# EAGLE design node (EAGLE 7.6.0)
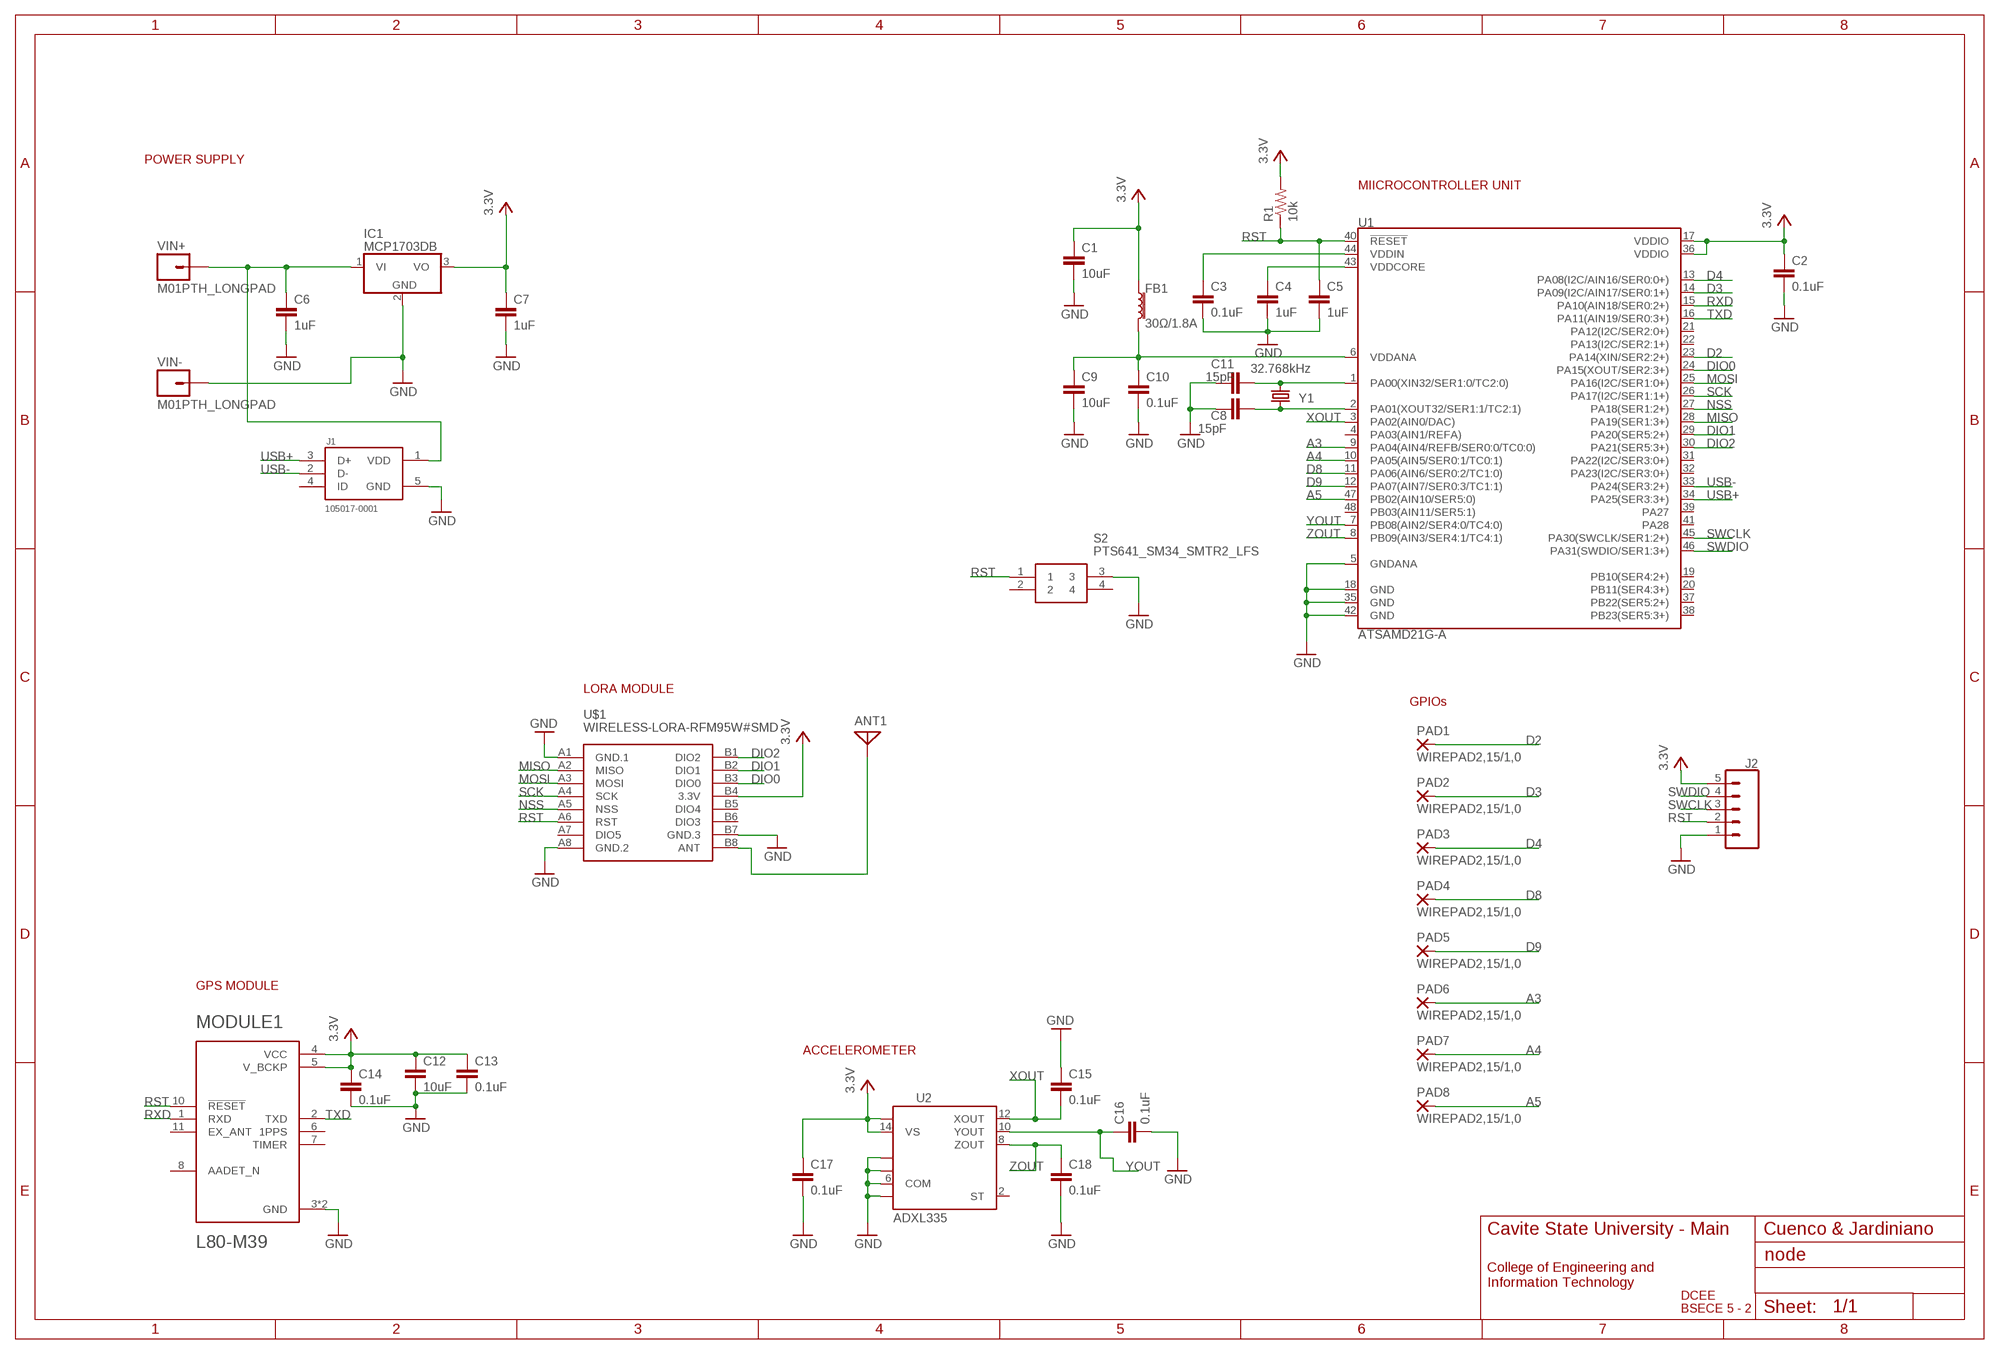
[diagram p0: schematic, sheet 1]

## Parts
ANT1  ANTENNA  [PAD-01]
C1  10uF  10UF-1206-6.3V-20%  [1206]
C2  0.1uF  10UF-1206-6.3V-20%  [1206]
C3  0.1uF  10UF-1206-6.3V-20%  [1206]
C4  1uF  10UF-1206-6.3V-20%  [1206]
C5  1uF  10UF-1206-6.3V-20%  [1206]
C6  1uF  10UF-1206-6.3V-20%  [1206]
C7  1uF  10UF-1206-6.3V-20%  [1206]
C8  15pF  10UF-1206-6.3V-20%  [1206]
C9  10uF  10UF-1206-6.3V-20%  [1206]
C10  0.1uF  10UF-1206-6.3V-20%  [1206]
C11  15pF  10UF-1206-6.3V-20%  [1206]
C12  10uF  10UF-1206-6.3V-20%  [1206]
C13  0.1uF  10UF-1206-6.3V-20%  [1206]
C14  0.1uF  10UF-1206-6.3V-20%  [1206]
C15  0.1uF  10UF-1206-6.3V-20%  [1206]
C16  0.1uF  10UF-1206-6.3V-20%  [1206]
C17  0.1uF  10UF-1206-6.3V-20%  [1206]
C18  0.1uF  10UF-1206-6.3V-20%  [1206]
FB1  30Ω/1.8A  FERRITE_BEAD-0603  [0603]
IC1  MCP1703DB  [SOT223]
J1  105017-0001  [MOLEX_105017-0001]
J2  CONN_05  [1X05]
MODULE1  L80-M39  [QUECTEL_L80-M39]
PAD1  WIREPAD2,15/1,0  [2,15/1,0]
PAD2  WIREPAD2,15/1,0  [2,15/1,0]
PAD3  WIREPAD2,15/1,0  [2,15/1,0]
PAD4  WIREPAD2,15/1,0  [2,15/1,0]
PAD5  WIREPAD2,15/1,0  [2,15/1,0]
PAD6  WIREPAD2,15/1,0  [2,15/1,0]
PAD7  WIREPAD2,15/1,0  [2,15/1,0]
PAD8  WIREPAD2,15/1,0  [2,15/1,0]
R1  10k  RESISTOR1206  [1206]
S2  PTS641_SM34_SMTR2_LFS  [PTS641_SM34]
U1  ATSAMD21G-A  [TQFP-48]
U2  ADXL335  [LFCSP-16]
U$1  WIRELESS-LORA-RFM95W#SMD  [WIRELESS-LORA-RFM95W#SMD]
VIN+  M01PTH_LONGPAD  [1X01_LONGPAD]
VIN-  M01PTH_LONGPAD  [1X01_LONGPAD]
Y1  32.768kHz  CRYSTAL-32.768KHZSMD-3.2X1.5  [CRYSTAL-SMD-3.2X1.5MM]

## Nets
A3: PAD6.1(P) U1.9(PA04(AIN4/REFB/SER0:0/TC0:0))
A4: PAD7.1(P) U1.10(PA05(AIN5/SER0:1/TC0:1))
A5: PAD8.1(P) U1.47(PB02(AIN10/SER5:0))
D2: PAD1.1(P) U1.23(PA14(XIN/SER2:2+))
D3: PAD2.1(P) U1.14(PA09(I2C/AIN17/SER0:1+))
D4: PAD3.1(P) U1.13(PA08(I2C/AIN16/SER0:0+))
D8: PAD4.1(P) U1.11(PA06(AIN6/SER0:2/TC1:0))
D9: PAD5.1(P) U1.12(PA07(AIN7/SER0:3/TC1:1))
DIO0: U1.24(PA15(XOUT/SER2:3+)) U$1.B3(DIO0)
DIO1: U1.29(PA20(SER5:2+)) U$1.B2(DIO1)
DIO2: U1.30(PA21(SER5:3+)) U$1.B1(DIO2)
FB1: C9.1 C10.1 FB1.2 U1.6(VDDANA)
GND: C1.2 C2.2 C3.2 C4.2 C5.2 C6.2 C7.2 C8.2 C9.2 C10.2 C11.1 C12.2 C13.2 C14.2 C15.1 C16.2 C17.2 C18.2 IC1.2(GND) J1.5(GND) J2.1 MODULE1.3(GND) MODULE1.12(GND) S2.3 U1.5(GNDANA) U1.18(GND) U1.35(GND) U1.42(GND) U2.3(COM) U2.5(COM) U2.6(COM) U2.7(COM) U$1.A1(GND.1) U$1.A8(GND.2) U$1.B7(GND.3) VIN-.1
MISO: U1.28(PA19(SER1:3+)) U$1.A2(MISO)
MOSI: U1.25(PA16(I2C/SER1:0+)) U$1.A3(MOSI)
N$1: C8.1 U1.1(PA00(XIN32/SER1:0/TC2:0)) Y1.P$2
N$2: C11.2 U1.2(PA01(XOUT32/SER1:1/TC2:1)) Y1.P$1
N$3: C4.1 U1.43(VDDCORE)
N$4: ANT1.1 U$1.B8(ANT)
N$5: C6.1 IC1.1(VI) J1.1(VDD) VIN+.1
N$6: C3.1 U1.44(VDDIN)
NSS: U1.27(PA18(SER1:2+)) U$1.A5(NSS)
RST: C5.1 J2.2 MODULE1.10(!RESET) R1.1 S2.1 U1.40(!RESET!) U$1.A6(RST)
RXD: MODULE1.1(RXD) U1.15(PA10(AIN18/SER0:2+))
SCK: U1.26(PA17(I2C/SER1:1+)) U$1.A4(SCK)
SWCLK: J2.3 U1.45(PA30(SWCLK/SER1:2+))
SWDIO: J2.4 U1.46(PA31(SWDIO/SER1:3+))
TXD: MODULE1.2(TXD) U1.16(PA11(AIN19/SER0:3+))
USB+: J1.3(D+) U1.34(PA25(SER3:3+))
USB-: J1.2(D-) U1.33(PA24(SER3:2+))
VCC: C1.1 C2.1 C7.1 C12.1 C13.1 C14.1 C17.1 FB1.1 IC1.3(VO) J2.5 MODULE1.4(VCC) MODULE1.5(V_BCKP) R1.2 U1.17(VDDIO) U1.36(VDDIO) U2.14(VS) U2.15(VS) U$1.B4(3.3V) ; supply symbol labelled 3.3V
XOUT: C15.2 U1.3(PA02(AIN0/DAC)) U2.12(XOUT)
YOUT: C16.1 U1.7(PB08(AIN2/SER4:0/TC4:0)) U2.10(YOUT)
ZOUT: C18.1 U1.8(PB09(AIN3/SER4:1/TC4:1)) U2.8(ZOUT)
Unconnected: J1.4(ID) MODULE1.6(1PPS) MODULE1.7(TIMER) MODULE1.8(AADET_N) MODULE1.11(EX_ANT) S2.2 S2.4 U1.4(PA03(AIN1/REFA)) U1.19(PB10(SER4:2+)) U1.20(PB11(SER4:3+)) U1.21(PA12(I2C/SER2:0+)) U1.22(PA13(I2C/SER2:1+)) U1.31(PA22(I2C/SER3:0+)) U1.32(PA23(I2C/SER3:0+)) U1.37(PB22(SER5:2+)) U1.38(PB23(SER5:3+)) U1.39(PA27) U1.41(PA28) U1.48(PB03(AIN11/SER5:1)) U2.2(ST) U$1.A7(DIO5) U$1.B5(DIO4) U$1.B6(DIO3)

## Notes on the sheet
- POWER SUPPLY
- MIICROCONTROLLER UNIT
- LORA MODULE
- GPIOs
- GPS MODULE
- ACCELEROMETER
- Cavite State University - Main | Cuenco & Jardiniano
- College of Engineering and
  Information Technology
- DCEE
- BSECE 5 - 2

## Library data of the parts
ANT1 = discrete:ANTENNA: Antenna
C1 C9 C12 = SparkFun-Capacitors:10UF: 10.0µF ceramic capacitors; PROD_ID: CAP-10057
C2-C8 C10 C11 C13-C18 = SparkFun-Capacitors:10UF: 10.0µF ceramic capacitors; PROD_ID: CAP-10057; VALUE: 10uF
FB1 = SparkFun-Coils:FERRITE_BEAD: Ferrite Bead (blocks, cores, rings, chokes, etc.); PROD_ID: NDUC-13805
IC1 = linear (1):MCP1703: 250 mA, 16V, Low Quiescent Current LDO Regulator Source: http://ww1.microchip.com/downloads/en/DeviceDoc/22049b.pdf
J1 = 105017-0001:105017-0001; AVAILABILITY: Unavailable; DESCRIPTION: Conn USB Type B M 5 POS 0.65mm Solder RA Thru-Hole 5 Terminal 1 Port Embossed T/R; MF: Molex, LLC; MP: 105017-0001; PACKAGE: None; PRICE: None
J2 = SparkFun-Connectors:CONN_05: Multi connection point. Often used as Generic Header-pin footprint for 0.1 inch spaced/style header connections On any of the 0.1 inch spaced packages, you can populate with these: Break Away Headers - Straight (PRT-00116) Break Away Male Headers - Right Angle (PRT-00553) Female Headers (PRT-00115)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
MODULE1 = L80-M39:L80-M39: GPS Receiver 1575.42MHz 3.3V 12-Pin; AVAILABILITY: Unavailable; DESCRIPTION: GPS Receiver 1575.42MHz 3.3V 12-Pin; MF: Quectel; MP: L80-M39; PACKAGE: None; PRICE: None
PAD1-PAD8 = wirepad:WIREPAD: Wire PAD connect wire on PCB
R1 = SparkFun:RESISTOR: Resistor
S2 = PTS641_SM34_SMTR2_LFS:PTS641_SM34_SMTR2_LFS: PTS641 Series SMT Top Actuated Switches Source: Datasheet; DESCRIPTION: PTS641 Series SMT Top Actuated Switches; HEIGHT: mm; MANUFACTURER_NAME: C & K COMPONENTS; MANUFACTURER_PART_NUMBER: PTS641 SM34 SMTR2 LFS; MOUSER_PART_NUMBER: 1359404P; MOUSER_PRICE-STOCK: http://uk.rs-online.com/web/p/products/1359404P; RS_PART_NUMBER: 1359404P; RS_PRICE-STOCK: http://uk.rs-online.com/web/p/products/1359404P
U1 = SparkFun-IC-Microcontroller:ATSAMD21G: Atmel SAMD21G SMART ARM-Based Microcontroller The Atmel ® | SMART ™ SAM D21 is a series of low-power microcontrollers using the 32-bit ARM ® Cortex ® -M0+ processor, and ranging from 32- to 64-pins with up to 256KB Flash and 32KB of SRAM. The SAM D21 devices operate at a maximum frequency of 48MHz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; PROD_ID: IC-13064
U2 = SparkFun:ADXL335
U$1 = diy-modules:WIRELESS-LORA-RFM95W: 868/915 MHz LoRa Radio Transceiver Module based on SX1276 chip Click here to find device on ebay.com
VIN+ VIN- = SparkFun:M01: Header 1
Y1 = SparkFun-Clocks:CRYSTAL-32.768KHZ: 32.768kHz Crystal; PROD_ID: XTAL-13062

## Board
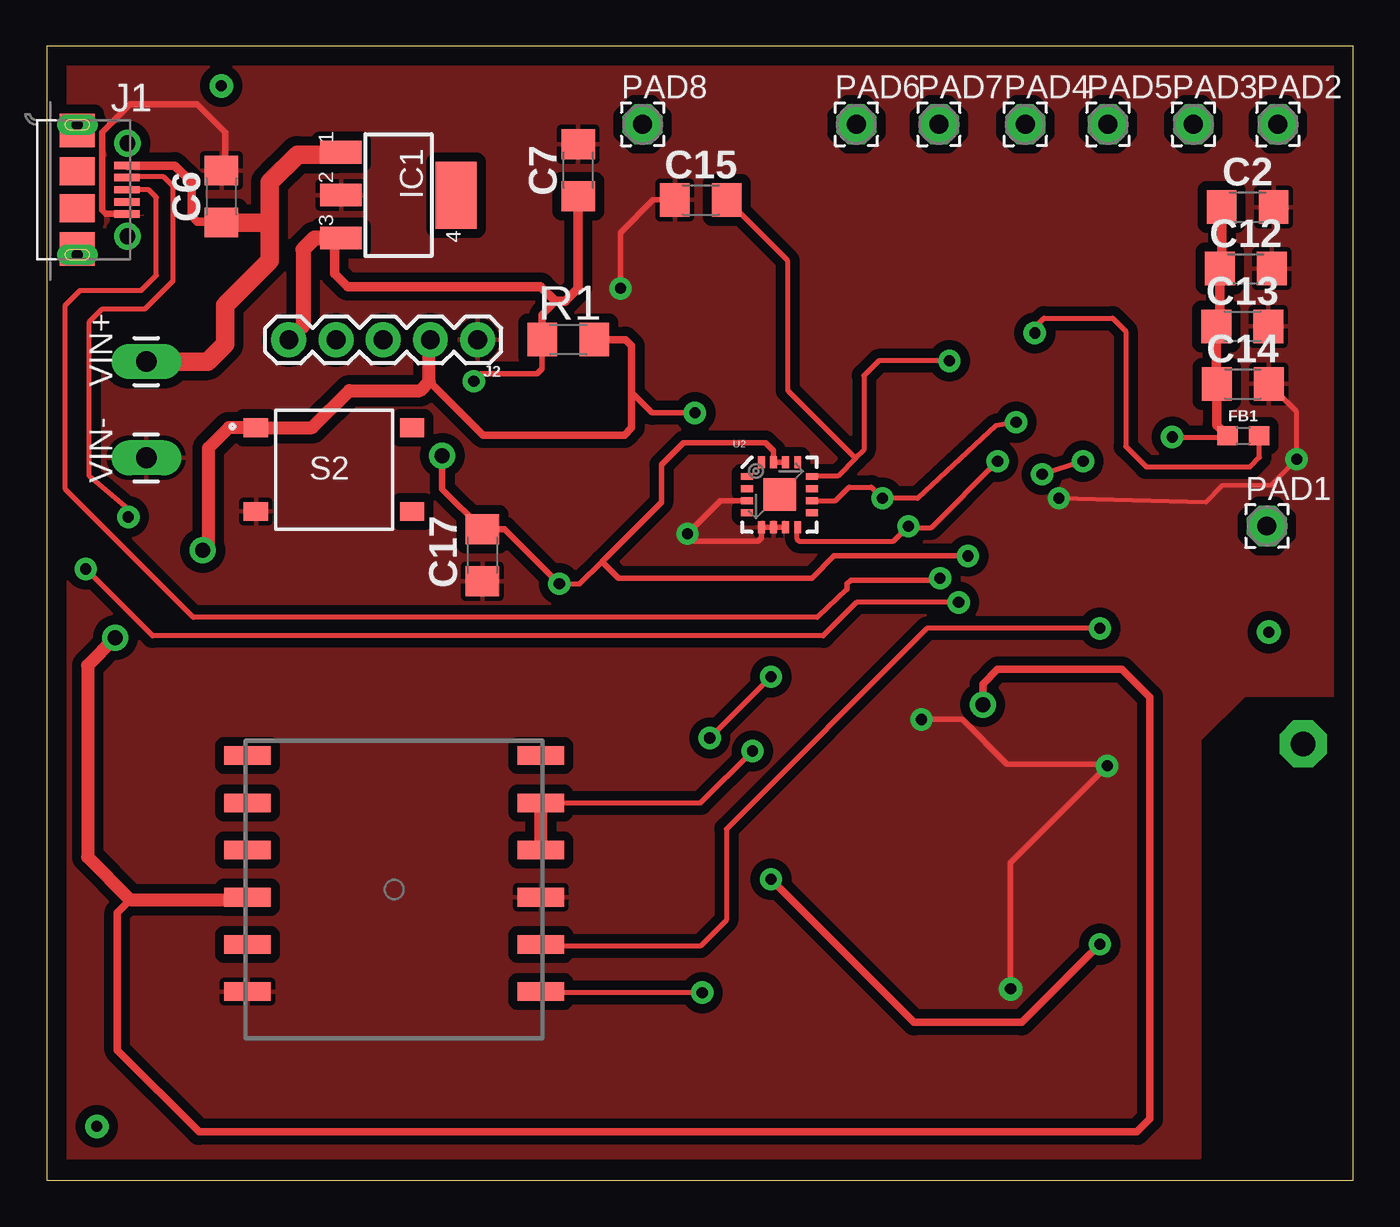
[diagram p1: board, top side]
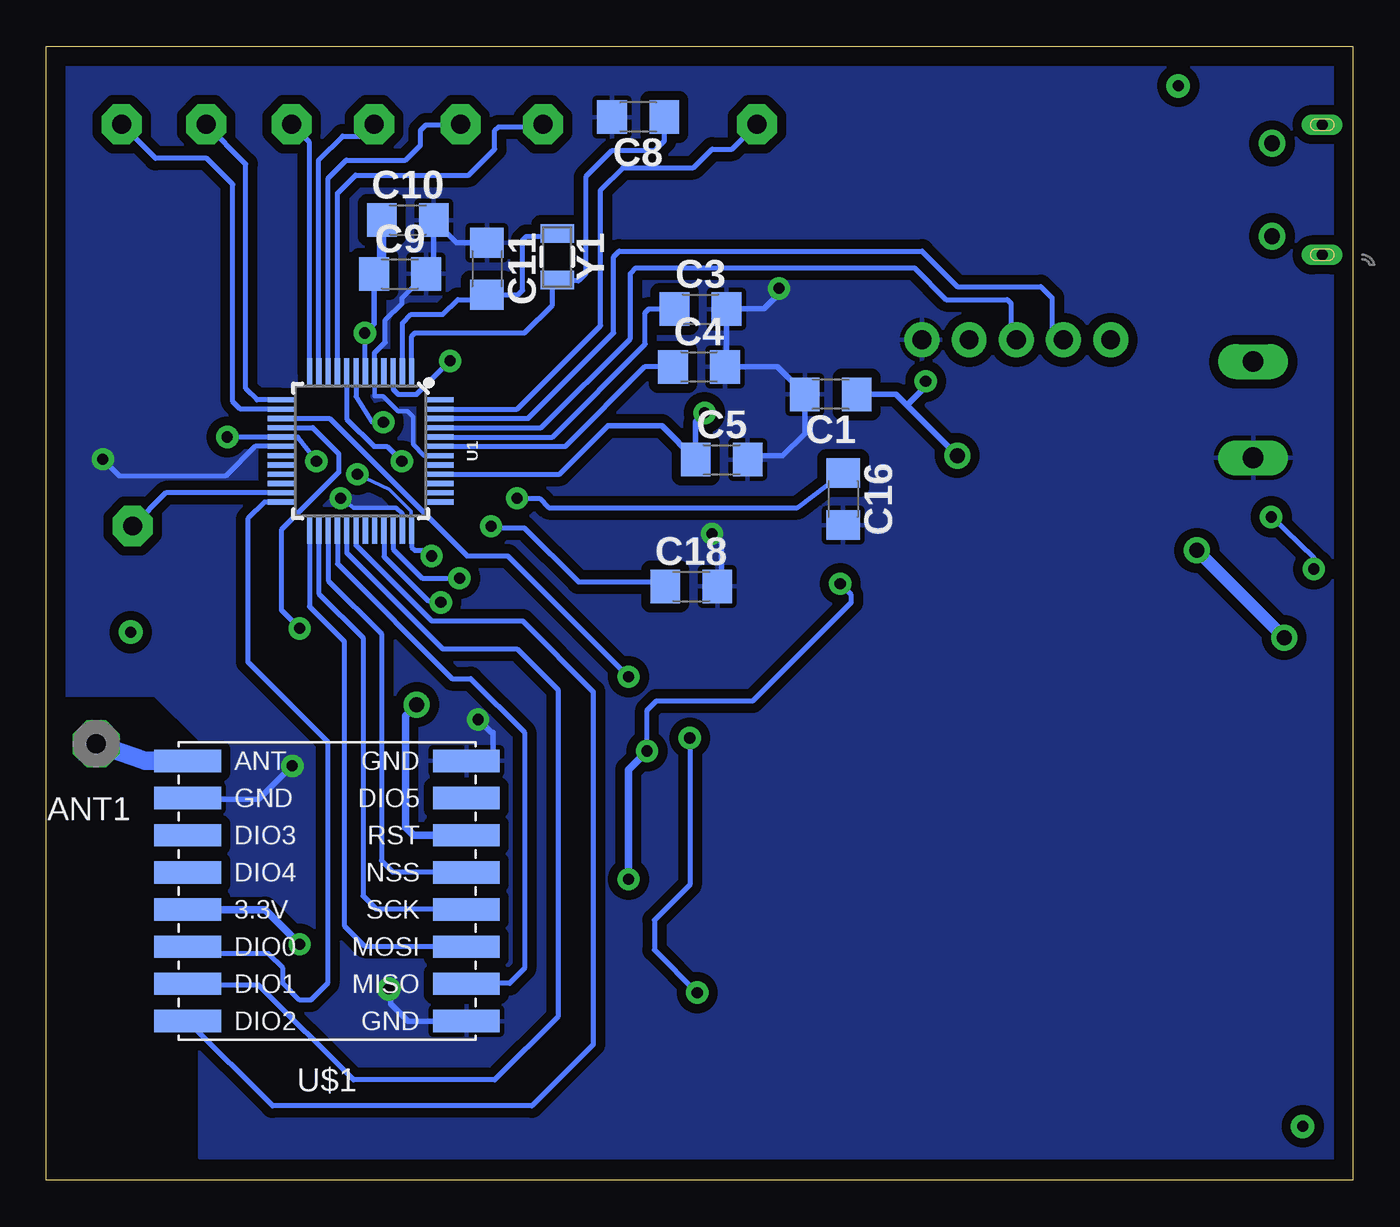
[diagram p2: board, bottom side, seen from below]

Size 70.34 x 61.02 mm. Coordinates in mm from the lower left corner, seen from the top.
Outline: 0,0 70.34,0 70.34,61.02 0,61.02 0,0
Copper layers (1*16): Top 0.035mm / dielectric 1.5mm / Bottom 0.035mm
Design rules "default *": minimum track width 4mil, minimum drill 16mil, track to track 8mil, track to pad 8mil, pad to pad 8mil, via to via 8mil, smd to smd 8mil, copper to edge 40mil, drill to drill 8mil, minimum pad ring 10mil, minimum via ring 8mil, stop-mask expansion 4mil, vias tented up to drill 0mil, thermal gap 10mil

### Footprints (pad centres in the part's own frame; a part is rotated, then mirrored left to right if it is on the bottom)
PAD-01 = drill 1.321 pad 2.54 octagon: 1 0,0
1206 = smd 1.6 x 1.8: 1 -1.4,0; 2 1.4,0
0603 = smd 1.1 x 1: 1 -0.85,0; 2 0.85,0
SOT223 = smd 1.219 x 2.235: 1 -2.311,-3.099; 2 0,-3.099; 3 2.311,-3.099 | smd 3.6 x 2.2: 4 0,3.099
MOLEX_105017-0001 = smd 0.4 x 1.35: 1 -1.3,2.675; 2 -0.65,2.675; 3 0,2.675; 4 0.65,2.675; 5 1.3,2.675 | drill 0.85 pad 1.45: P$1 -2.5,2.7; P$2 2.5,2.7 | smd 1.5 x 1.9: P$8 -1,0; P$9 1,0 | smd 1.8 x 1.9: P$10 -3.2,0; P$11 3.2,0 | drill 0.6 pad 0.8 long: P$12 -3.5,0; P$13 3.5,0
1X05 = drill 1.016 pad 1.88: 1 0,0; 2 2.54,0; 3 5.08,0; 4 7.62,0; 5 10.16,0
QUECTEL_L80-M39 = smd 2.5 x 1: 1 7.9,-5.5; 2 7.9,-2.96; 3 7.9,-0.42; 4 7.9,2.12; 5 7.9,4.66; 6 7.9,7.2; 7 -7.9,7.2; 8 -7.9,4.66; 9 -7.9,2.12; 10 -7.9,-0.42; 11 -7.9,-2.96; 12 -7.9,-5.5
2,15/1,0 = drill 1.016 pad 2.159 octagon: 1 0,0
PTS641_SM34 = smd 1.3 x 1: 1 -4.2,2.25; 2 4.2,2.25; 3 -4.2,-2.25; 4 4.2,-2.25
TQFP-48 = smd 1.5 x 0.28: 1 -4.25,2.75; 2 -4.25,2.25; 3 -4.25,1.75; 4 -4.25,1.25; 5 -4.25,0.75; 6 -4.25,0.25; 7 -4.25,-0.25; 8 -4.25,-0.75; 9 -4.25,-1.25; 10 -4.25,-1.75; 11 -4.25,-2.25; 12 -4.25,-2.75; 25 4.25,-2.75; 26 4.25,-2.25; 27 4.25,-1.75; 28 4.25,-1.25; 29 4.25,-0.75; 30 4.25,-0.25; 31 4.25,0.25; 32 4.25,0.75; 33 4.25,1.25; 34 4.25,1.75; 35 4.25,2.25; 36 4.25,2.75 | smd 0.28 x 1.5: 13 -2.75,-4.25; 14 -2.25,-4.25; 15 -1.75,-4.25; 16 -1.25,-4.25; 17 -0.75,-4.25; 18 -0.25,-4.25; 19 0.25,-4.25; 20 0.75,-4.25; 21 1.25,-4.25; 22 1.75,-4.25; 23 2.25,-4.25; 24 2.75,-4.25; 37 2.75,4.25; 38 2.25,4.25; 39 1.75,4.25; 40 1.25,4.25; 41 0.75,4.25; 42 0.25,4.25; 43 -0.25,4.25; 44 -0.75,4.25; 45 -1.25,4.25; 46 -1.75,4.25; 47 -2.25,4.25; 48 -2.75,4.25
LFCSP-16 = smd 1.75 x 1.75: 0 0,0 | smd 0.65 x 0.37: 1 -1.75,0.975; 2 -1.75,0.325; 3 -1.75,-0.325; 4 -1.75,-0.975; 9 1.75,-0.975; 10 1.75,-0.325; 11 1.75,0.325; 12 1.75,0.975 | smd 0.37 x 0.65: 5 -0.975,-1.75; 6 -0.325,-1.75; 7 0.325,-1.75; 8 0.975,-1.75; 13 0.975,1.75; 14 0.325,1.75; 15 -0.325,1.75; 16 -0.975,1.75
WIRELESS-LORA-RFM95W#SMD = smd 3.6 x 1.2: A1 -7.5,7; A2 -7.5,5; A3 -7.5,3; A4 -7.5,1; A5 -7.5,-1; A6 -7.5,-3; A7 -7.5,-5; A8 -7.5,-7; B1 7.5,7; B2 7.5,5; B3 7.5,3; B4 7.5,1; B5 7.5,-1; B6 7.5,-3; B7 7.5,-5; B8 7.5,-7
1X01_LONGPAD = drill 1.118 pad 1.88 long: 1 0,0
CRYSTAL-SMD-3.2X1.5MM = smd 1 x 1.8: P$1 -1.25,0; P$2 1.25,0

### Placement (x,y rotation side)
ANT1  67.65,23.49 180 bottom
C1  28.11,42.3 180 bottom
C2  64.66,52.38 0 top
C3  35.12,46.88 0 bottom
C4  35.2,43.78 0 bottom
C5  33.98,38.78 0 bottom
C6  9.42,52.94 90 top
C7  28.62,54.36 90 top
C8  38.48,57.22 180 bottom
C9  51.3,48.78 0 bottom
C10  50.88,51.68 0 bottom
C11  46.62,49.06 270 bottom
C12  64.56,49.06 0 top
C13  64.38,45.96 0 top
C14  64.4,42.86 0 top
C15  35.22,52.76 0 top
C16  27.44,36.66 270 bottom
C17  23.46,33.64 270 top
C18  35.62,31.96 0 bottom
FB1  64.42,40.07 0 top
IC1  18.94,53.02 270 top
J1  1.65,53.31 270 top
J2  23.2,45.23 180 top
MODULE1  18.71,15.65 0 top
PAD1  65.7,35.21 0 top
PAD2  66.29,56.83 0 top
PAD3  61.74,56.83 0 top
PAD4  52.69,56.83 0 top
PAD5  57.14,56.83 0 top
PAD6  43.59,56.83 0 top
PAD7  48.04,56.83 0 top
PAD8  32.09,56.83 0 top
R1  28.08,45.24 180 top
S2  15.47,38.25 0 top
U1  53.42,39.25 270 bottom
U2  39.46,36.9 0 top
U$1  55.23,15.57 180 bottom
VIN+  5.37,44.06 90 top
VIN-  5.37,38.88 90 top
Y1  42.84,49.7 270 bottom

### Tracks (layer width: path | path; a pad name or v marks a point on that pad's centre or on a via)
A3
  Bottom 0.279: U1.9 54.67,53.13 53.7,54.1 47.6,54.1 46.2,55.5 46.2,56.5 46,56.7 43.72,56.7 PAD6.1
A4
  Bottom 0.279: U1.10 55.17,53.93 54.2,54.9 51,54.9 50.2,55.7 50.2,56.5 49.9,56.8 48.07,56.8 PAD7.1
A5
  Bottom 0.279: U1.47 45,41.5 40.5,46 40.5,53.3 39.3,54.5 35.5,54.5 34.5,55.5 33.42,55.5 PAD8.1
D2
  Bottom 0.279: U1.23 63.91,37 PAD1.1
D3
  Bottom 0.279: U1.14 59.9,41.5 60.3,41.9 60.3,53.6 61.7,55 64.46,55 PAD2.1
D4
  Bottom 0.279: U1.13 59,42 59.6,42.6 59.6,54.69 PAD3.1
D8
  Bottom 0.279: U1.11 55.67,54.93 54.4,56.2 53.32,56.2 PAD4.1
D9
  Bottom 0.279: U1.12 56.17,55.86 PAD5.1
DIO0
  Bottom 0.279: U1.24 58.6,36.5 59.5,35.6 59.5,27.9 55.2,23.6 55.2,10.6 56.1,9.7 56.7,9.7 57.6,10.6 57.6,11.4 58.4,12.2 62.36,12.2 U$1.B3
DIO1
  Bottom 0.279: U1.29 54.17,33.77 49,28.6 45,28.6 42.8,26.4 42.8,8.8 46.2,5.4 53.8,5.4 58.9,10.5 62.66,10.5 U$1.B2
DIO2
  Bottom 0.279: U1.30 53.67,34.17 49.6,30.1 44.7,30.1 40.9,26.3 40.9,7.3 44.2,4 58.16,4 U$1.B1
FB1  (via drill 0.6 pad 1.2)
  Top 0.279: v53.2,45.6 53.2,45.9 53.7,46.4 57.4,46.4 58.1,45.7 58.1,39.5 59.2,38.4 64.8,38.4 65.3,38.9 65.3,40.04 FB1.2
  Bottom 0.279: U1.6 53.17,45.57 v53.2,45.6
  Bottom 0.3: C9.1 52.7,46.1 v53.2,45.6
  Bottom 0.5: C10.1 52.28,49.2 C9.1
GND  (via drill 0.6 pad 1.2, 0.6 pad 1.27)
  Top 0.25: v54.5,36.7 62.4,36.5 63.3,37.4 65.9,37.4 v67.3,38.8
  Top 0.279: v67.3,38.8 67.3,41.36 C14.2
  Top 0.3: U2.7 U2.6 U2.5 38.48,34.59 38.3,34.4 34.9,34.4 v34.5,34.8 36.27,36.58 U2.3 | C15.1 32.66,52.76 30.9,51 v30.9,48 | v47.1,24.8 49.3,24.8 51.7,22.4 57,22.4 v57.1,22.3 51.9,17.1 v51.9,10.3
  Top 0.35: J1.5 3.19,52.01 3,52.2 3,56.4 4.5,57.9 8.1,57.9 9.6,56.4 9.6,54.52 C6.2
  Bottom 0.25: U1.42 50,39 50.6,39.6 50.6,41.1 50.9,41.4 51.4,41.4 52.2,42.2 52.67,42.2 U1.5 | U1.35 51.17,35.87 51.5,36.2 53.8,36.2 v54.5,36.7
  Bottom 0.279: U1.5 52.67,44.53 52.1,45.1 52.1,46.3 51.2,47.2 51.2,47.48 C9.2 | U1.18 59.1,39.5 60.7,37.9 66.4,37.9 v67.3,38.8
  Bottom 0.3: C9.2 49.48,49.2 C10.2 48.26,50.46 C11.1 | v34.5,34.8 34,34.3 34,32.18 C18.2 | C5.2 32.36,39 30.7,39 29.51,40.19 C1.2 30.99,43.78 C4.2 33.72,43.86 C3.2 33.7,46.9 31.7,46.9 30.9,47.7 v30.9,48 | U$1.A8 46.3,22.57 46.3,24.1 46.4,24.1 v47.1,24.8 | v57.1,22.3 58.9,20.5 62.66,20.5 U$1.B7 | U$1.A1 50.87,8.57 51.8,9.5 51.8,10.2 v51.9,10.3
  pour Top (isolate 0.5): 0.9,60.3 69.6,60.3 69.6,26.1 64.5,26.1 62.1,23.7 62.1,1.2 0.9,1.2
  pour Bottom (isolate 0.5): 0.9,60.3 69.6,60.3 69.6,26.1 64.5,26.1 62.1,23.7 62.1,1.2 0.9,1.2
MISO
  Bottom 0.279: U1.28 54.67,33.17 48.5,27 47.5,27 44.6,24.1 44.6,11.4 45.4,10.6 47.7,10.6 U$1.A2
MOSI
  Bottom 0.279: U1.25 56.17,30.87 54.3,29 54.3,13.7 53.2,12.6 47.76,12.6 U$1.A3
N$1
  Bottom 0.279: U1.1 50.67,45.43 50.5,45.6 44.6,45.6 43.1,47.1 43.1,48.19 Y1.P$2 42.79,48.4 41.7,48.4 41.3,48.8 41.3,54 39.9,55.4 37.6,55.4 37.08,55.92 C8.1
N$2
  Bottom 0.279: U1.2 51.17,46.13 50.7,46.6 49,46.6 48.2,47.4 46.98,47.4 C11.2 44.94,47.66 44.7,47.9 44.7,50.6 44.5,50.8 42.99,50.8 Y1.P$1
N$3
  Bottom 0.279: U1.43 42.4,39.5 38.1,43.8 36.62,43.8 C4.1
N$4
  Bottom 1: U$1.B8 65.03,22.57 ANT1.1
N$5
  Top 0.45: J1.1 6.89,54.61 7.8,53.7 7.8,51.9 8.1,51.6 9.36,51.6 C6.1
  Top 1: VIN+.1 8.66,44.06 9.6,45 9.6,47.1 12,49.5 12,51.6 | 12,51.6 12,53.7 13.5,55.2 15.71,55.2 IC1.1 | C6.1 11.94,51.54 12,51.6
N$6
  Bottom 0.279: U1.44 43.1,40 38.1,45 38.1,46.7 37.9,46.9 36.54,46.9 C3.1
N$7  (via drill 0.6 pad 1.27)
  other vias: 2.7,2.9
N$8  (via drill 0.6 pad 1.27)
  other vias: 9.4,58.9
N$14  (via drill 0.6 pad 1.27)
  other vias: 65.8,29.5
NSS
  Bottom 0.279: U1.27 55.17,32.27 52.3,29.4 52.3,17.2 51.7,16.6 47.76,16.6 U$1.A5
RST  (via drill 0.6 pad 1.2, 0.8 pad 1.4)
  Top 0.3: v34.9,41.3 32.6,41.3 31.5,42.4
  Top 0.4: v50.4,25.6 50.4,26.7 51.2,27.5 57.9,27.5 59.4,26 59.4,3.3 58.7,2.6 8.2,2.6 3.8,7 3.8,14.4 4.5,15.1 | R1.1 31.16,45.24 31.5,44.9 31.5,42.4 31.5,40.5 31.1,40.1 23.5,40.1 20.6,43
  Top 0.7: J2.2 20.6,45.17 20.6,43 20.1,42.5 16.3,42.5 14.3,40.5 S2.1 9.8,40.5 8.7,39.4 8.7,34.2 v8.4,33.9 | v3.7,29.2 2.2,27.7 2.2,17.4 4.5,15.1 10.68,15.1 MODULE1.10
  Bottom 0.279: U1.40 42.7,38 40.1,40.6
  Bottom 0.3: 40.1,40.6 37.2,40.6 C5.1 35.38,40.82 v34.9,41.3
  Bottom 0.4: U$1.A6 50.57,18.57 51,19 51,25 v50.4,25.6
  Bottom 0.7: v8.4,33.9 v3.7,29.2
RXD  (via drill 0.6 pad 1.2)
  Top 0.279: 26.46,10.3 MODULE1.1 | 26.56,10.1 MODULE1.1 | v35.3,10.1 26.66,10.1 MODULE1.1 | v39,27.1 v35.7,23.8
  Bottom 0.279: U1.15 55.1,41 47.7,33.6 45.5,33.6 v39,27.1 | v35.7,23.8 35.7,15.9 37.6,14 37.6,12.4 v35.3,10.1
SCK
  Bottom 0.279: U1.26 55.67,31.57 53.3,29.2 53.3,15.3 52.6,14.6 47.76,14.6 U$1.A4
SWCLK
  Bottom 0.279: U1.45 43.7,40.5 38.9,45.3 38.9,48.8 38.6,49.1 23.6,49.1 21.9,47.4 18.6,47.4 18.4,47.2 18.4,45.51 J2.3
SWDIO
  Bottom 0.279: U1.46 44.4,41 39.8,45.6 39.8,49.7 39.5,50 23.2,50 21.3,48.1 16.8,48.1 16.2,47.5 16.2,45.85 J2.4
TXD  (via drill 0.6 pad 1.2)
  Top 0.279: v56.7,29.7 47.4,29.7 36.6,18.9 36.6,14 35.2,12.6 26.7,12.6 MODULE1.2
  Bottom 0.279: U1.16 56,40.5 54.6,39.1 54.6,38.1 57.7,35 57.7,30.7 v56.7,29.7
USB+  (via drill 0.6 pad 1.2)
  Top 0.279: 43.1,31.8 41.5,30.3 7.9,30.3 1,37.2 1,47.1 1.8,47.9 5.1,47.9 5.9,48.7 5.9,52.9 5.5,53.3 4.33,53.3 J1.3
  Top 0.3: 43.1,31.8 43.1,32.1 43.3,32.3 48,32.3 v48.1,32.4
  Bottom 0.279: U1.34 51.67,33.97 50.1,32.4 v48.1,32.4
USB-  (via drill 0.6 pad 1.2)
  Top 0.279: v2.1,32.9 5.7,29.3 41.8,29.3 43.6,31.1 v49.1,31.1 | v4.4,35.7 4.4,36.1 2.3,37.9 2.3,46.2 3,46.9 5.3,46.9 6.8,48.4 6.8,53.5 6.3,54 4.37,54 J1.2
  Bottom 0.279: U1.33 52.17,33.57 49.8,31.2 49.2,31.2 v49.1,31.1 | v2.1,32.9 2.1,33.5 v4.4,35.7
VCC  (via drill 0.6 pad 1.2, 0.8 pad 1.4)
  Top 0.279: v60.6,40 63.5,40 FB1.1 | MODULE1.5 35.21,20.31 v38,23.1 | v27.6,32.1 28.7,32.1 | v55.8,38.7 v53.6,38
  Top 0.3: U2.14 U2.15 39.13,39.27 38.7,39.7 34.3,39.7 33.1,38.5 33.1,36.5 29.9,33.3 | 29.9,33.3 28.7,32.1 | v49.6,33.6 42.4,33.6 41.2,32.4 30.8,32.4 29.9,33.3 | R1.2 26.68,43.68 26.4,43.4 23.4,43.4 v23,43
  Top 0.35: v21.3,39 21.3,37.2 C17.1 24.66,35.04 v27.6,32.1
  Top 0.4: v56.7,12.7 52.5,8.5 46.7,8.5 v39,16.2 | R1.2 26.68,46.58 27.4,47.3
  Top 0.5: C2.1 63.26,49.16 C12.1 63.16,46.14 C13.1 62.98,42.88 C14.1 63,40.64 FB1.1 | C7.1 28.62,48.02 27.9,47.3 27.4,47.3 26.6,48.1 16.2,48.1 15.5,48.8 15.5,50.37 IC1.3
  Top 0.7: MODULE1.4 MODULE1.5
  Top 0.8: IC1.3 14.41,50.71 13.8,50.1 13.8,45.99 J2.5
  Bottom 0.2: v53.6,38 51.9,37.2 50.7,36 50.7,35.03 U1.36
  Bottom 0.279: U1.36 50.67,34.07 50.5,33.9 49.9,33.9 v49.6,33.6 | v60.6,40 U1.17 56.8,40 v55.8,38.7 | v38,23.1 38,25.3 37.5,25.8 32.3,25.8 27,31.1 27,31.5 v27.6,32.1
  Bottom 0.3: 24,41.7 24.6,42.3 C1.1 | 24,41.7 v21.3,39 | v23,43 23,42.7 24,41.7
  Bottom 0.4: U$1.B4 58.57,14.57 v56.7,12.7 | v39,16.2 39,22.1 v38,23.1
XOUT  (via drill 0.6 pad 1.2)
  Top 0.279: v48.6,44.1 44.8,44.1 44,43.3 44,39.3 43.55,38.85 | 43.55,38.85 42.6,37.9 41.23,37.9 U2.12 | 43.55,38.85 39.9,42.5 39.9,49.48 C15.2
  Bottom 0.279: U1.3 51.67,42.57 51.4,42.3 50.4,42.3 v48.6,44.1
YOUT  (via drill 0.6 pad 1.2)
  Top 0.279: v52.2,40.8 51.1,40.6 46.9,36.7 v45,36.7 44.4,37.3 43.2,37.3 42.48,36.58 U2.10 41.23,36.6
  Bottom 0.279: U1.7 53.67,42.17 52.8,40.8 v52.2,40.8 | v45,36.7 43.8,36.7 43.3,36.2 29.9,36.2 C16.1
ZOUT  (via drill 0.6 pad 1.2)
  Top 0.279: U2.8 40.4,35.12 40.4,34.5 40.5,34.4 45.6,34.4 v46.4,35.2 46.5,35.1 47.6,35.1 v51.2,38.7
  Bottom 0.279: U1.8 54.17,40.97 52.7,39.5 52,39.5 v51.2,38.7 | C18.1 37.26,32.2 41.7,32.2 44.6,35.1 46.3,35.1 v46.4,35.2

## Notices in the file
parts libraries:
SparkFun: Licensing: CC v3.0 Share-Alike You are welcome to use this library for commercial purposes.
SparkFun-Capacitors: Licensing: Creative Commons ShareAlike 4.0 International - https://creativecommons.org/licenses/by-sa/4.0
